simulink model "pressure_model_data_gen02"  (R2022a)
settings: Solver=VariableStepAuto  StartTime=0.0  StopTime=tfin  RelTol=1e-3
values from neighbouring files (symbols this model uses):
  Ts = 5    [sisopres.m]

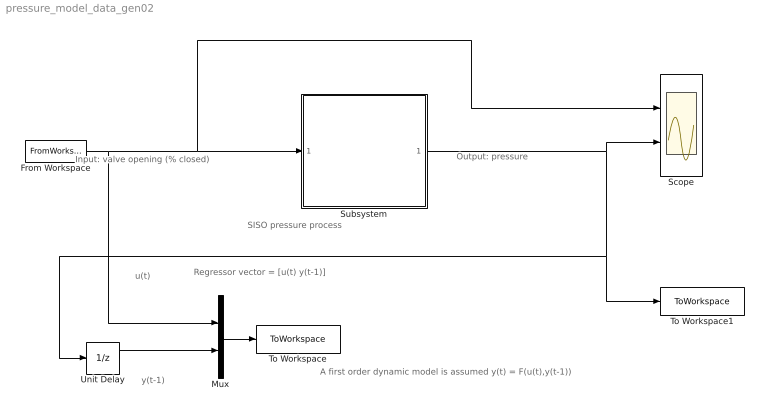
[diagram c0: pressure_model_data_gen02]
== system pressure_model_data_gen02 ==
  note: Regressor vector = [u(t) y(t-1)]
  note: y(t-1)
  note: u(t)
  note: A first order dynamic model is assumed y(t) = F(u(t),y(t-1))
  note: Output: pressure
  note: Input: valve opening (% closed)
  note: SISO pressure process
  From Workspace : FromWorkspace  VariableName=[tsim U]  SampleTime=Ts
  Mux : Mux  Inputs=2
  Scope : Scope  NumInputPorts=2
  Subsystem : Subsystem
  To Workspace : ToWorkspace  VariableName=Psim  SampleTime=Ts
  To Workspace1 : ToWorkspace  VariableName=Tsim  SampleTime=Ts
  Unit Delay : UnitDelay  SampleTime=Ts  HasFrameUpgradeWarning=on
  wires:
  From Workspace/1 -> Mux/1, Scope/1, Subsystem/1(u)
  Subsystem/1(y) -> Unit Delay/1, To Workspace1/1, Scope/2
  Mux/1 -> To Workspace/1
  Unit Delay/1 -> Mux/2

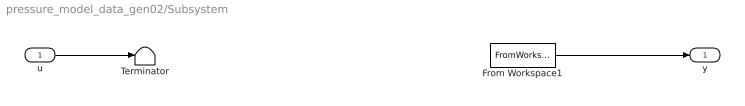
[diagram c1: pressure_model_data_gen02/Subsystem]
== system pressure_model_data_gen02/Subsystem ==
  u : Inport
  From Workspace1 : FromWorkspace  VariableName=[tsim Y]  SampleTime=Ts
  Terminator : Terminator
  y : Outport
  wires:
  From Workspace1/1 -> y/1
  u/1 -> Terminator/1
